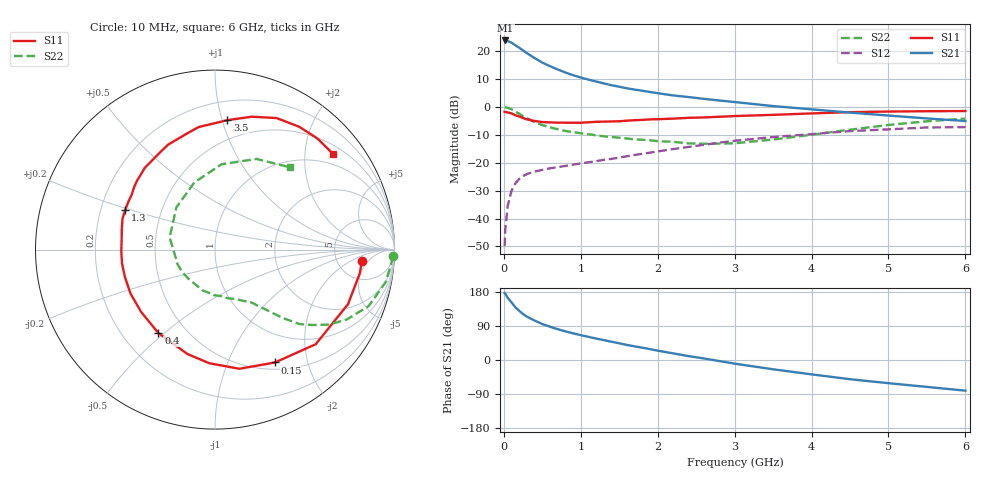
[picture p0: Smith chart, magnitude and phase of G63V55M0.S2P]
! SIEMENS Small Signal Semiconductors
! BFG193
! Si NPN RF Bipolar Junction Transistor in SOT223
! VCE = 3.5 V  IC = 5 mA
! Common Emitter S-Parameters:  August  1996
# GHz  S  MA  R  50
!  f  S11  S21  S12  S22
! GHz  MAG  ANG  MAG  ANG  MAG  ANG  MAG  ANG
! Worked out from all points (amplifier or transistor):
!   36 points, 10 MHz to 6 GHz, reference 50 ohm
!   highest |S21| = 23.9 dB at 20 MHz (marker M1)
!   |S21| within 3 dB of that: start of sweep to 220.1 MHz
!   unconditionally stable (mu >= 1): 1.102 GHz to 2.552 GHz
!   at 250 MHz: K = 0.34, MSG = 22.5 dB, |S12| = -24.8 dB
!   at 1.4 GHz: K = 1.09, MAG = 11.4 dB, |S12| = -18.6 dB
!   at 6 GHz: K = 0.88, MSG = 1.1 dB, |S12| = -7.2 dB
!   S11 on the Smith chart (normalised r, x): 10 MHz: 8.71, -3.51; 150 MHz: 0.59, -1.50; 400 MHz: 0.35, -0.48; 1.3 GHz: 0.30, +0.19; 3.5 GHz: 0.34, +1.04; 6 GHz: 0.70, +2.66
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0.01  0.8205 -4.6  15.57 176.7  0.0032 93.5  0.9912 -2.2
0.02  0.8178 -9.2  15.62 174.5  0.0067 87.3  0.9855 -4.3
0.05  0.8011 -22.3  15.2 164.3  0.0167 77.4  0.9688 -10.7
0.1  0.77 -43.2  14.24 151.9  0.0315 68.8  0.9121 -20.2
0.15  0.7122 -62.0  12.79 139.0  0.0428 60.2  0.8305 -28.0
0.2  0.6776 -78.5  11.57 129.9  0.0514 54.5  0.7592 -33.4
0.25  0.6337 -92.9  10.34 121.2  0.0577 49.3  0.6841 -37.9
0.3  0.6016 -104.8  9.248 114.5  0.0629 46.1  0.6288 -41.3
0.4  0.5617 -124.2  7.537 104.1  0.0697 41.8  0.536 -45.3
0.5  0.5385 -139.9  6.269 94.9  0.0748 39.1  0.4748 -47.9
0.6  0.5306 -152.5  5.401 87.8  0.0797 38.3  0.4317 -50.1
0.7  0.5246 -163.1  4.717 81.3  0.0836 38.1  0.3999 -52.3
0.9  0.5221 -179.2  3.725 70.3  0.0929 38.0  0.3535 -55.9
1.1  0.5321 167.4  3.101 61.0  0.1021 38.7  0.3245 -61.5
1.3  0.5471 156.2  2.652 52.4  0.1131 39.0  0.2983 -66.9
1.6  0.5695 142.3  2.167 39.7  0.1311 38.2  0.2729 -78.2
2.2  0.6196 120.4  1.615 17.5  0.1761 33.3  0.238 -106.6
2.8  0.6691 102.5  1.311 -2.8  0.2296 24.4  0.2212 -144.9
3.5  0.7244 84.5  1.04 -24.5  0.2893 9.5  0.2616 165.0
4.5  0.8093 64.9  0.795 -50.7  0.3703 -11.2  0.392 107.0
5.5  0.8417 47.4  0.625 -71.0  0.4299 -37.1  0.5556 65.4
6  0.8472 39.0  0.561 -80.9  0.4362 -51.8  0.6203 47.6
